| TEXAS INSTRUMENTS INCORPORATED
| Standard Linear and Logic Group
| IBIS Model of SN74ALVCH16269
| 12-BIT TO 24-BIT REGISTERED BUS EXCHANGER WITH 3-STATE OUTPUTS
| This file contains package information for the following:
|  TSSOP 56-pin (DGG) package as [Component] ALVCH16269_DGG
|  SSOP 56-pin (DL) package as [Component] ALVCH16269_DL
|  VFBGA 56-PIN (GQL) PACKAGE AS [COMPONENT] ALVCH16269_GQL
| This device can be powered at the following Vccs:
|  1.8 volt Vcc
|  2.5 volt Vcc
|  3.3 volt Vcc
| This file provides unique models under the [Model Selector] for each Vcc.
| For operation at a specific Vcc, select the appropriate model after each
| [Model Selector] keyword.
[IBIS Ver]   3.2
[Comment char]  |_char
[File Name]   sn74alvch16269.ibs
[File Rev]   1.1 | b_die
[Date]   May 12, 2004
[Source]   Data created from TI-SPICE simulations at TI-SLL.
[Notes]   The following is an IBIS list for the ALVCH16269.
   Please contact sllibis@ti.com with questions and
   comments concerning SLL IBIS models.
   - FILE REV HISTORY
   - 1.1 Release IBIS file on 05/13/04
   - Non-monotonic data in ground-clamp due to bus-hold
[Disclaimer] Property of Texas Instruments Incorporated.  Unauthorized
   reproduction and/or distribution is strictly prohibited.
   This product is protected under copyright law.
   Created  2004, (C) Copyright  2004, Texas Instruments
   Incorporated, All Rights Reserved
   UNLESS THERE IS A SIGNED, WRITTEN AGREEMENT TO THE
   CONTRARY, TEXAS INSTRUMENTS (TI) IS PROVIDING THE IBIS
   MODELS  AND WITHOUT ANY WARRANTY, EXPRESSED OR
   IMPLIED.  TI assumes no liability for:
   1) the accuracy of the IBIS models provided to your
   company;
   2) the proper functioning of these IBIS Models in your
   design or for any resulting applications; or
   3) infringement of patents, copyrights or intellectual
   property rights resulting from your use of these IBIS
   models.
   TI provides IBIS Models as a service to our customers.
   You and your company shall not distribute, sell or give
   these models to anyone else without prior written
   permission from TI.
   TI reserves the right to make changes to our products or
   to discontinue any semiconductor product or service
   without notice, and advises our customers to obtain the
   latest version of relevant information to verify, before
   placing orders, that the information being relied on is
   current.
   Please be aware that your receipt and use of the IBIS
   information provided shall serve as acceptance of these
   terms and conditions.  If you do not accept these terms,
   you should return or destroy the IBIS models and any
   other accompanying information immediately.
| Component ALVCH16269_DGG 56-pin TSSOP
[Component]   ALVCH16269_DGG
[Manufacturer]   Texas Instruments, Inc.
[Package]
|   typ   min   max
R_pkg   4.500e-02   3.500e-02   6.200e-02
L_pkg   3.324e-09   2.403e-09   5.094e-09
C_pkg   5.640e-13   3.410e-13   9.140e-13
[Pin]   signal_name   model_name   R_pin   L_pin   C_pin
1   OEA   ALVCH16269_OE   6.200e-02   5.094e-09   8.560e-13
2   OEB1   ALVCH16269_OE   6.100e-02   4.621e-09   9.020e-13
3   2B3   ALVCH16269_IO   6.000e-02   4.316e-09   8.020e-13
4   GND   GND   5.900e-02   3.968e-09   6.980e-13
5   2B2   ALVCH16269_IO   5.700e-02   3.716e-09   6.490e-13
6   2B1   ALVCH16269_IO   4.200e-02   3.517e-09   6.530e-13
7   VCC   POWER   4.100e-02   3.160e-09   5.700e-13
8   A1   ALVCH16269_IO   3.900e-02   2.981e-09   4.820e-13
9   A2   ALVCH16269_IO   3.900e-02   2.808e-09   4.470e-13
10   A3   ALVCH16269_IO   3.800e-02   2.715e-09   4.090e-13
11   GND   GND   4.100e-02   2.675e-09   3.910e-13
12   A4   ALVCH16269_IO   3.900e-02   2.536e-09   3.660e-13
13   A5   ALVCH16269_IO   3.900e-02   2.457e-09   3.480e-13
14   A6   ALVCH16269_IO   3.800e-02   2.411e-09   3.530e-13
15   A7   ALVCH16269_IO   3.900e-02   2.456e-09   3.550e-13
16   A8   ALVCH16269_IO   3.900e-02   2.471e-09   3.490e-13
17   A9   ALVCH16269_IO   4.000e-02   2.580e-09   3.700e-13
18   GND   GND   3.800e-02   2.651e-09   3.890e-13
19   A10   ALVCH16269_IO   3.800e-02   2.739e-09   4.110e-13
20   A11   ALVCH16269_IO   3.900e-02   2.838e-09   4.490e-13
21   A12   ALVCH16269_IO   3.800e-02   2.988e-09   4.840e-13
22   VCC   POWER   3.800e-02   3.104e-09   5.640e-13
23   1B1   ALVCH16269_IO   4.000e-02   3.427e-09   6.380e-13
24   1B2   ALVCH16269_IO   5.600e-02   3.654e-09   6.410e-13
25   GND   GND   5.700e-02   3.932e-09   7.000e-13
26   1B3   ALVCH16269_IO   5.800e-02   4.257e-09   8.060e-13
27   NC   NC   5.700e-02   4.580e-09   9.140e-13
28   SELECT   ALVCH16269_SEL   5.900e-02   5.038e-09   8.610e-13
29   CLK   ALVCH16269_CLK   6.000e-02   5.058e-09   8.580e-13
30   CENA1   ALVCH16269_CLK   5.600e-02   4.543e-09   9.040e-13
31   1B4   ALVCH16269_IO   5.700e-02   4.241e-09   8.020e-13
32   GND   GND   5.900e-02   3.933e-09   6.990e-13
33   1B5   ALVCH16269_IO   5.600e-02   3.616e-09   6.370e-13
34   1B6   ALVCH16269_IO   3.700e-02   3.368e-09   6.400e-13
35   VCC   POWER   3.600e-02   3.024e-09   5.630e-13
36   1B7   ALVCH16269_IO   3.500e-02   2.876e-09   4.740e-13
37   1B8   ALVCH16269_IO   3.500e-02   2.745e-09   4.440e-13
38   1B9   ALVCH16269_IO   3.700e-02   2.683e-09   4.050e-13
39   GND   GND   3.800e-02   2.603e-09   3.820e-13
40   1B10   ALVCH16269_IO   3.800e-02   2.510e-09   3.620e-13
41   1B11   ALVCH16269_IO   3.600e-02   2.412e-09   3.410e-13
42   1B12   ALVCH16269_IO   3.800e-02   2.416e-09   3.490e-13
43   2B12   ALVCH16269_IO   3.800e-02   2.403e-09   3.490e-13
44   2B11   ALVCH16269_IO   3.700e-02   2.429e-09   3.410e-13
45   2B10   ALVCH16269_IO   3.600e-02   2.483e-09   3.580e-13
46   GND   GND   3.700e-02   2.614e-09   3.810e-13
47   2B9   ALVCH16269_IO   3.500e-02   2.669e-09   4.020e-13
48   2B8   ALVCH16269_IO   3.600e-02   2.763e-09   4.420e-13
49   2B7   ALVCH16269_IO   3.600e-02   2.942e-09   4.780e-13
50   VCC   POWER   3.500e-02   3.053e-09   5.640e-13
51   2B6   ALVCH16269_IO   3.600e-02   3.408e-09   6.410e-13
52   2B5   ALVCH16269_IO   5.800e-02   3.698e-09   6.410e-13
53   GND   GND   5.900e-02   3.974e-09   6.970e-13
54   2B4   ALVCH16269_IO   6.100e-02   4.327e-09   8.020e-13
55   CENA2   ALVCH16269_CLK   6.100e-02   4.624e-09   9.050e-13
56   OEB2   ALVCH16269_OE   6.000e-02   5.063e-09   8.580e-13
| Component ALVCH16269_DL 56-pin SSOP
[Component]   ALVCH16269_DL
[Manufacturer]   Texas Instruments, Inc.
[Package]
|   typ   min   max
R_pkg   5.500e-02   4.800e-02   6.700e-02
L_pkg   6.539e-09   4.803e-09   9.746e-09
C_pkg   8.570e-13   5.000e-13   1.351e-12
[Pin]   signal_name   model_name   R_pin   L_pin   C_pin
1   OEA   ALVCH16269_OE   6.400e-02   9.646e-09   1.202e-12
2   OEB1   ALVCH16269_OE   5.900e-02   8.723e-09   1.348e-12
3   2B3   ALVCH16269_IO   5.900e-02   8.139e-09   1.223e-12
4   GND   GND   5.600e-02   7.554e-09   1.088e-12
5   2B2   ALVCH16269_IO   5.400e-02   6.991e-09   9.660e-13
6   2B1   ALVCH16269_IO   5.300e-02   6.659e-09   9.730e-13
7   VCC   POWER   5.500e-02   6.321e-09   9.050e-13
8   A1   ALVCH16269_IO   5.600e-02   5.942e-09   7.130e-13
9   A2   ALVCH16269_IO   5.700e-02   5.768e-09   6.780e-13
10   A3   ALVCH16269_IO   5.400e-02   5.459e-09   6.310e-13
11   GND   GND   5.100e-02   5.224e-09   6.380e-13
12   A4   ALVCH16269_IO   4.800e-02   5.088e-09   6.010e-13
13   A5   ALVCH16269_IO   5.000e-02   5.021e-09   5.180e-13
14   A6   ALVCH16269_IO   5.100e-02   4.803e-09   5.000e-13
15   A7   ALVCH16269_IO   5.100e-02   4.803e-09   5.000e-13
16   A8   ALVCH16269_IO   5.000e-02   5.021e-09   5.180e-13
17   A9   ALVCH16269_IO   4.800e-02   5.088e-09   6.010e-13
18   GND   GND   5.100e-02   5.224e-09   6.380e-13
19   A10   ALVCH16269_IO   5.400e-02   5.459e-09   6.310e-13
20   A11   ALVCH16269_IO   5.700e-02   5.768e-09   6.770e-13
21   A12   ALVCH16269_IO   5.500e-02   5.942e-09   7.150e-13
22   VCC   POWER   5.500e-02   6.321e-09   9.070e-13
23   1B1   ALVCH16269_IO   5.300e-02   6.659e-09   9.720e-13
24   1B2   ALVCH16269_IO   5.400e-02   6.991e-09   9.660e-13
25   GND   GND   5.600e-02   7.554e-09   1.087e-12
26   1B3   ALVCH16269_IO   5.900e-02   8.139e-09   1.223e-12
27   NC   NC   5.900e-02   8.727e-09   1.351e-12
28   SELECT   ALVCH16269_SEL   6.700e-02   9.746e-09   1.210e-12
29   CLK   ALVCH16269_CLK   6.300e-02   9.630e-09   1.203e-12
30   CENA1   ALVCH16269_CLK   6.000e-02   8.751e-09   1.349e-12
31   1B4   ALVCH16269_IO   6.000e-02   8.184e-09   1.224e-12
32   GND   GND   5.600e-02   7.543e-09   1.087e-12
33   1B5   ALVCH16269_IO   5.400e-02   7.005e-09   9.690e-13
34   1B6   ALVCH16269_IO   5.600e-02   6.714e-09   9.750e-13
35   VCC   POWER   5.800e-02   6.384e-09   9.090e-13
36   1B7   ALVCH16269_IO   5.700e-02   5.976e-09   7.170e-13
37   1B8   ALVCH16269_IO   5.700e-02   5.743e-09   6.770e-13
38   1B9   ALVCH16269_IO   5.400e-02   5.468e-09   6.310e-13
39   GND   GND   5.500e-02   5.329e-09   6.440e-13
40   1B10   ALVCH16269_IO   5.200e-02   5.189e-09   6.060e-13
41   1B11   ALVCH16269_IO   5.200e-02   5.053e-09   5.190e-13
42   1B12   ALVCH16269_IO   5.200e-02   4.825e-09   5.020e-13
43   2B12   ALVCH16269_IO   5.400e-02   4.897e-09   5.060e-13
44   2B11   ALVCH16269_IO   5.200e-02   5.093e-09   5.210e-13
45   2B10   ALVCH16269_IO   5.100e-02   5.179e-09   6.080e-13
46   GND   GND   5.400e-02   5.314e-09   6.450e-13
47   2B9   ALVCH16269_IO   5.500e-02   5.511e-09   6.320e-13
48   2B8   ALVCH16269_IO   5.700e-02   5.770e-09   6.770e-13
49   2B7   ALVCH16269_IO   5.600e-02   5.956e-09   7.160e-13
50   VCC   POWER   5.500e-02   6.320e-09   9.050e-13
51   2B6   ALVCH16269_IO   5.200e-02   6.621e-09   9.680e-13
52   2B5   ALVCH16269_IO   5.300e-02   6.974e-09   9.660e-13
53   GND   GND   5.700e-02   7.571e-09   1.089e-12
54   2B4   ALVCH16269_IO   5.700e-02   8.097e-09   1.219e-12
55   CENA2   ALVCH16269_CLK   5.900e-02   8.723e-09   1.349e-12
56   OEB2   ALVCH16269_OE   6.100e-02   9.560e-09   1.199e-12
|   VFBGA PACKAGE (GQL)
[Component]   ALVCH16269_GQL
[manufacturer]   Texas Instruments, Inc.
[Package]
|   typ   min   max
R_pkg   0.065   0.035   0.097
L_pkg   1.952nH   1.000nH   3.191nH
C_pkg   0.283pF   0.162pF   0.434pF
[Pin] signal_name   model_name   R_pin   L_pin   C_pin
A3   OEA   ALVCH16269_OE   0.036   1.004nH   0.176pF
A2   OEB1   ALVCH16269_OE   0.04   1.191nH   0.186pF
A1   2B3   ALVCH16269_IO   0.047   1.411nH   0.209pF
B3   GND   GND   0.097   3.191nH   0.434pF
B2   2B2   ALVCH16269_IO   0.074   2.213nH   0.329pF
B1   2B1   ALVCH16269_IO   0.06   1.712nH   0.243pF
C3   VCC   POWER   0.085   2.691nH   0.368pF
C2   A1   ALVCH16269_IO   0.074   2.16nH   0.315pF
C1   A2   ALVCH16269_IO   0.06   1.666nH   0.247pF
D2   A3   ALVCH16269_IO   0.074   2.121nH   0.313pF
D3   GND   GND   0.091   2.924nH   0.397pF
D1   A4   ALVCH16269_IO   0.06   1.619nH   0.245pF
E2   A5   ALVCH16269_IO   0.069   2.031nH   0.288pF
E1   A6   ALVCH16269_IO   0.06   1.583nH   0.22pF
F1   A7   ALVCH16269_IO   0.06   1.578nH   0.22pF
F2   A8   ALVCH16269_IO   0.069   2.017nH   0.286pF
G1   A9   ALVCH16269_IO   0.06   1.594nH   0.241pF
G3   GND   GND   0.092   2.917nH   0.397pF
G2   A10   ALVCH16269_IO   0.075   2.114nH   0.315pF
H1   A11   ALVCH16269_IO   0.06   1.632nH   0.247pF
H2   A12   ALVCH16269_IO   0.07   2.074nH   0.307pF
H3   VCC   POWER   0.086   2.664nH   0.365pF
J1   1B1   ALVCH16269_IO   0.06   1.689nH   0.249pF
J2   1B2   ALVCH16269_IO   0.066   2.152nH   0.332pF
J3   GND   GND   0.087   3.118nH   0.423pF
K1   1B3   ALVCH16269_IO   0.038   1.303nH   0.2pF
K2   NC   NC   0.035   1.176nH   0.183pF
K3   SELECT   ALVCH16269_SEL   0.035   1.007nH   0.162pF
K4   CLK   ALVCH16269_CLK   0.035   1.000nH   0.162pF
K5   CENA1   ALVCH16269_CLK   0.035   1.154nH   0.18pF
K6   1B4   ALVCH16269_IO   0.041   1.352nH   0.204pF
J4   GND   GND   0.088   3.137nH   0.43pF
J5   1B5   ALVCH16269_IO   0.074   2.218nH   0.334pF
J6   1B6   ALVCH16269_IO   0.06   1.683nH   0.25pF
H4   VCC   POWER   0.085   2.658nH   0.372pF
H5   1B7   ALVCH16269_IO   0.075   2.149nH   0.321pF
H6   1B8   ALVCH16269_IO   0.06   1.627nH   0.248pF
G5   1B9   ALVCH16269_IO   0.075   2.113nH   0.314pF
G4   GND   GND   0.092   2.922nH   0.396pF
G6   1B10   ALVCH16269_IO   0.06   1.594nH   0.242pF
F5   1B11   ALVCH16269_IO   0.069   2.016nH   0.288pF
F6   1B12   ALVCH16269_IO   0.06   1.58nH   0.221pF
E6   2B12   ALVCH16269_IO   0.06   1.582nH   0.22pF
E5   2B11   ALVCH16269_IO   0.069   2.026nH   0.289pF
D6   2B10   ALVCH16269_IO   0.06   1.61nH   0.245pF
D4   GND   GND   0.092   2.933nH   0.396pF
D5   2B9   ALVCH16269_IO   0.075   2.126nH   0.311pF
C6   2B8   ALVCH16269_IO   0.06   1.641nH   0.245pF
C5   2B7   ALVCH16269_IO   0.073   2.168nH   0.319pF
C4   VCC   POWER   0.086   2.675nH   0.362pF
B6   2B6   ALVCH16269_IO   0.06   1.688nH   0.243pF
B5   2B5   ALVCH16269_IO   0.075   2.281nH   0.333pF
B4   GND   GND   0.095   3.168nH   0.424pF
A6   2B4   ALVCH16269_IO   0.045   1.418nH   0.209pF
A5   CENA2   ALVCH16269_CLK   0.039   1.216nH   0.19pF
A4   OEB2   ALVCH16269_OE   0.037   1.029nH   0.179pF
| Model ALVCH16269_CLK
[Model Selector]   ALVCH16269_CLK
ALVCH16269_CLK_18   1.8 volt Vcc
ALVCH16269_CLK_25   2.5 volt Vcc
ALVCH16269_CLK_33   3.3 volt Vcc
| Model ALVCH16269_OE
[Model Selector]   ALVCH16269_OE
ALVCH16269_OE_18   1.8 volt Vcc
ALVCH16269_OE_25   2.5 volt Vcc
ALVCH16269_OE_33   3.3 volt Vcc
| Model ALVCH16269_SEL
[Model Selector]   ALVCH16269_SEL
ALVCH16269_SEL_18   1.8 volt Vcc
ALVCH16269_SEL_25   2.5 volt Vcc
ALVCH16269_SEL_33   3.3 volt Vcc
| Model ALVCH16269_IO
[Model Selector]   ALVCH16269_IO
ALVCH16269_IO_18   1.8 volt Vcc
ALVCH16269_IO_25   2.5 volt Vcc
ALVCH16269_IO_33   3.3 volt Vcc
| Models and submodels in the file (12): ALVCH16269_CLK_18 (Input), ALVCH16269_CLK_25 (Input), ALVCH16269_CLK_33 (Input), ALVCH16269_OE_18 (Input), ALVCH16269_OE_25 (Input), ALVCH16269_OE_33 (Input), ALVCH16269_SEL_18 (Input), ALVCH16269_SEL_25 (Input), ALVCH16269_SEL_33 (Input), ALVCH16269_IO_18 (3-state), ALVCH16269_IO_25 (3-state), ALVCH16269_IO_33 (3-state)
